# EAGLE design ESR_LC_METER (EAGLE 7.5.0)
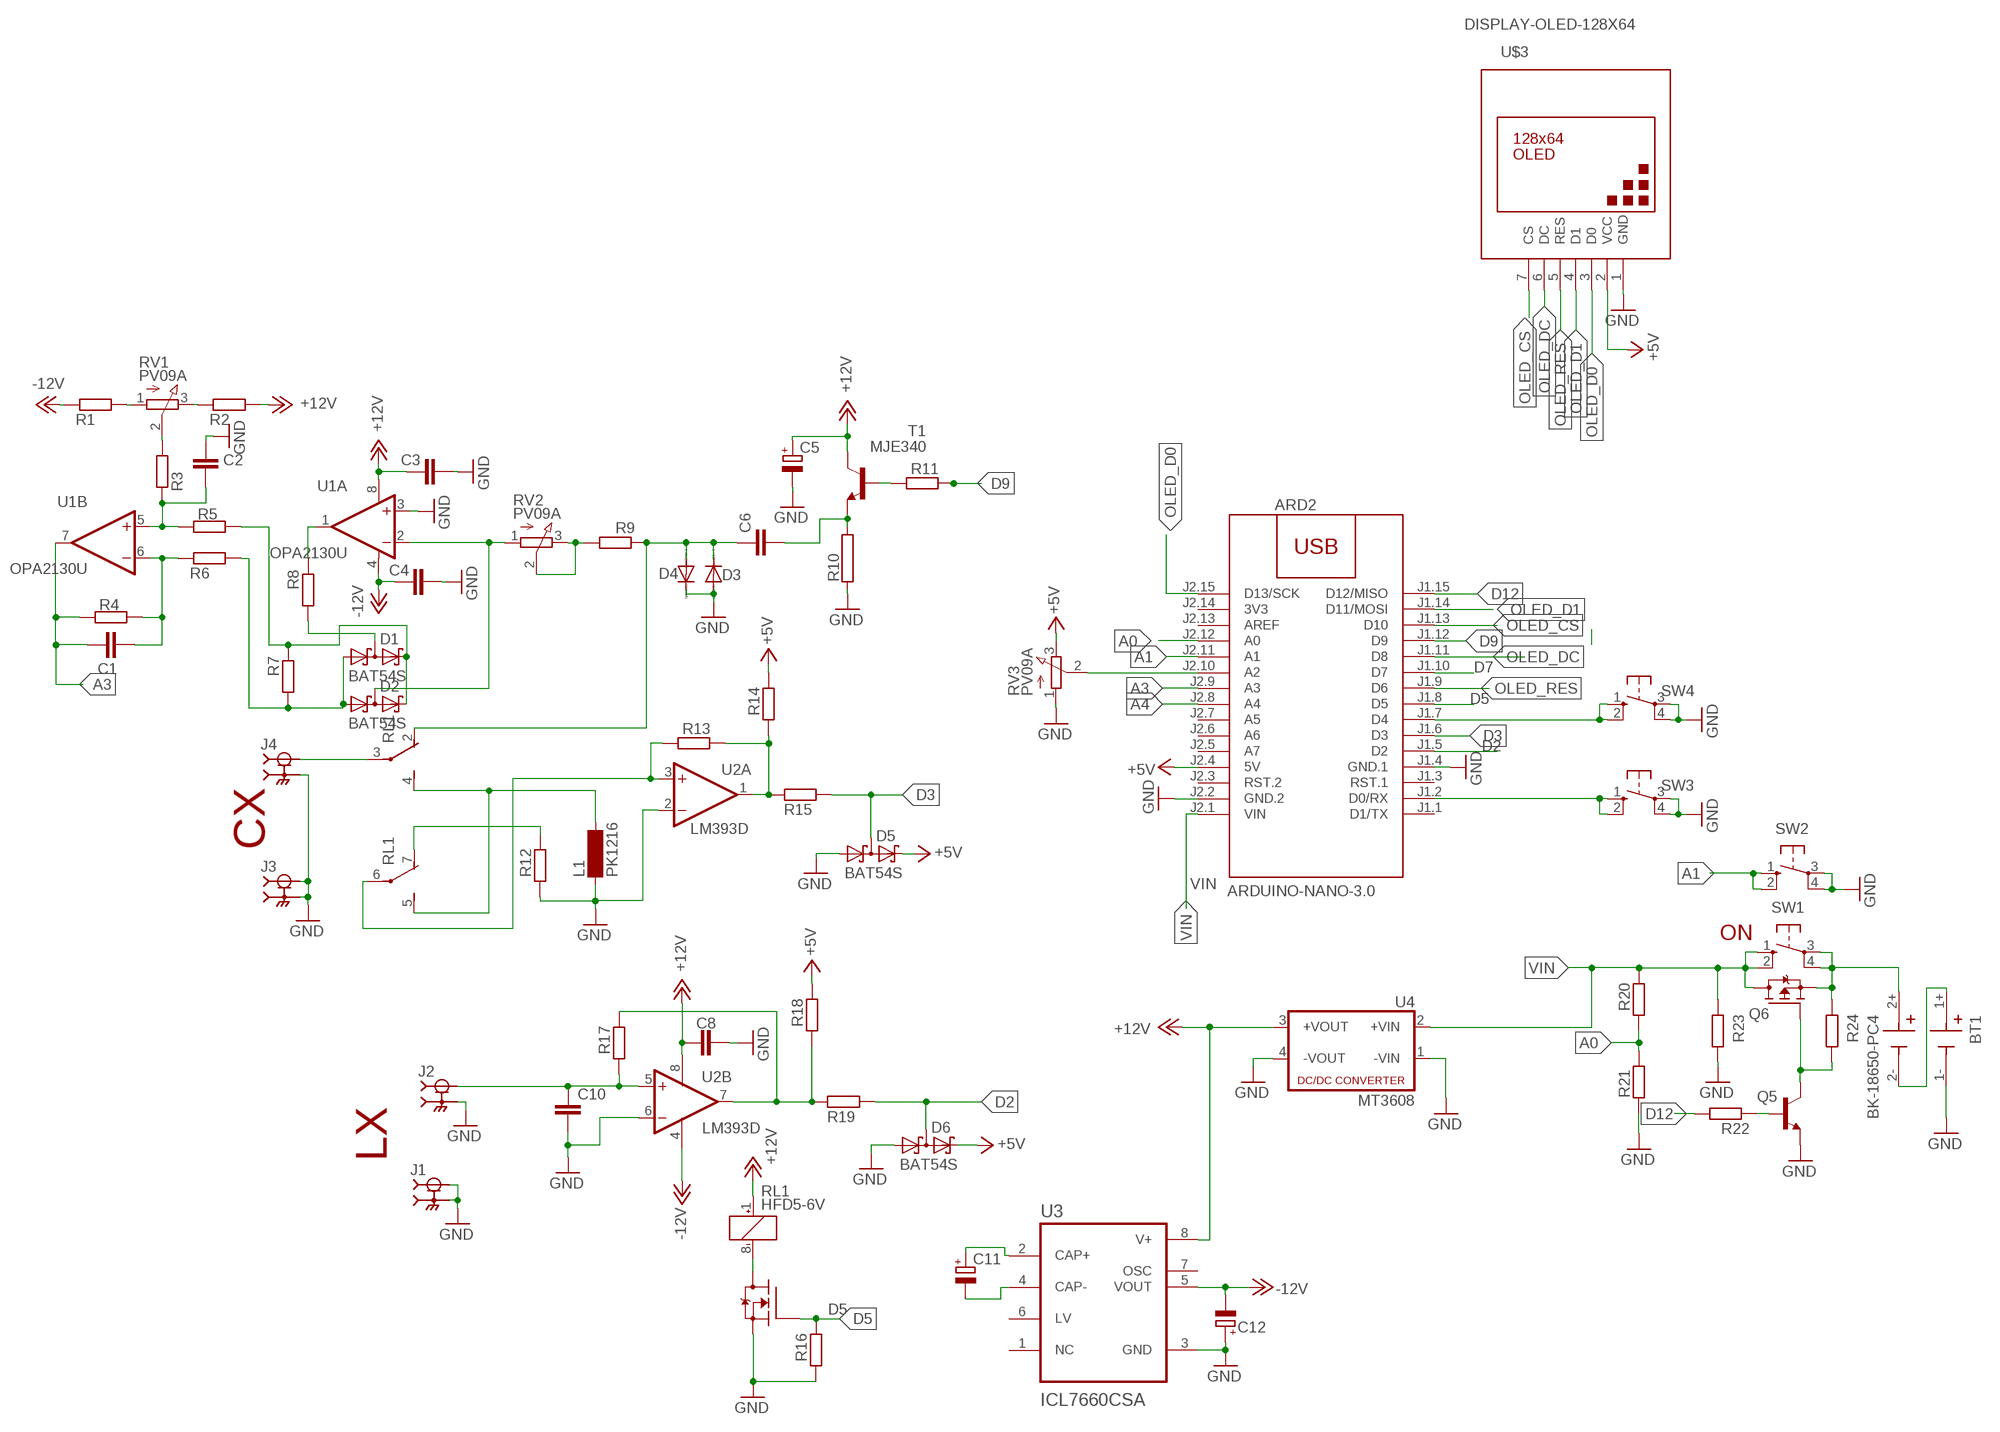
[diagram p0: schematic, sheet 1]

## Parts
ARD2  ARDUINO-NANO-3.0  [ARDUINO-NANO-3.0]
BT1  BK-18650-PC4  [BAT_BK-18650-PC4]
C1  C-EUC0805  [C0805]
C2  C-EUC0805  [C0805]
C3  C-EUC0805  [C0805]
C4  C-EUC0805  [C0805]
C5  CPOL-EUSMCA  [SMC_A]
C6  C-EUC0805  [C0805]
C8  C-EUC0805  [C0805]
C10  C-EUC1206  [C1206]
C11  CPOL-EUSMCA  [SMC_A]
C12  CPOL-EUSMCA  [SMC_A]
D1  BAT54S  [SOT23]
D2  BAT54S  [SOT23]
D3  1N4004  [DO41-10]
D4  1N4004  [DO41-10]
D5  BAT54S  [SOT23]
D6  BAT54S  [SOT23]
J1  BNC7T-J-P-XX-RA-BH1  [SAMTEC_BNC7T-J-P-XX-RA-BH1]
J2  BNC7T-J-P-XX-RA-BH1  [SAMTEC_BNC7T-J-P-XX-RA-BH1]
J3  BNC7T-J-P-XX-RA-BH1  [SAMTEC_BNC7T-J-P-XX-RA-BH1]
J4  BNC7T-J-P-XX-RA-BH1  [SAMTEC_BNC7T-J-P-XX-RA-BH1]
L1  PK1216  BS11  [BS11]
Q3  ZVN3310F  [SOT23]
Q5  BC817-16LT1SMD  [SOT23-BEC]
Q6  STR2P3LLH6  [SOT23]
R1  R-EU_R0805  [R0805]
R2  R-EU_R0805  [R0805]
R3  R-EU_R0805  [R0805]
R4  R-EU_R0805  [R0805]
R5  R-EU_R0805  [R0805]
R6  R-EU_R0805  [R0805]
R7  R-EU_R0805  [R0805]
R8  R-EU_R0805  [R0805]
R9  R-EU_R0805  [R0805]
R10  RAC04  [AC04]
R11  R-EU_R0805  [R0805]
R12  R-EU_R0805  [R0805]
R13  R-EU_R0805  [R0805]
R14  R-EU_R0805  [R0805]
R15  R-EU_R0805  [R0805]
R16  R-EU_R0805  [R0805]
R17  R-EU_R0805  [R0805]
R18  R-EU_R0805  [R0805]
R19  R-EU_R0805  [R0805]
R20  R-EU_R0805  [R0805]
R21  R-EU_R0805  [R0805]
R22  R-EU_R0805  [R0805]
R23  R-EU_R0805  [R0805]
R24  R-EU_R0805  [R0805]
RL1  HFD5-6V  G6J-2P-Y  [G6J-2P-Y]
RV1  PV09A  [PTV09]
RV2  PV09A  [PTV09]
RV3  PV09A  [PTV09]
SW1  10-XX  [B3F-10XX]
SW2  10-XX  [B3F-10XX]
SW3  10-XX  [B3F-10XX]
SW4  10-XX  [B3F-10XX]
T1  MJE340  [TO126]
U1  OPA2130U  [SO08]
U2  LM393D  [SO08]
U3  ICL7660CSA  [SOIC127P600X175-8N]
U4  MT3608  [MT3608]
U$3  DISPLAY-OLED-128X64  [DISPLAY-OLED-128X64]

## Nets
+5V: ARD2.J2.4(5V) D5.2(C2) D6.2(C2) R14.2 R18.2 RV3.3(E) U$3.2(VCC)
+12V: C3.1 C5.+ C8.1 R2.1 RL1.1(1:+) T1.2(C) U1.8(A:V+) U2.8(P:V+) U3.8(V+) U4.3(+VOUT)
-12V: C4.1 C12.- R1.2 U1.4(A:V-) U2.4(P:V-) U3.5(VOUT)
A0: ARD2.J2.12(A0) R20.1 R21.2
A1: ARD2.J2.11(A1) SW2.1(S) SW2.2(S1)
A3: ARD2.J2.9(A3) C1.2 R4.2 U1.7(B:OUT)
A4: ARD2.J2.8(A4)
BAT: BT1.2+ Q6.3(S) R24.2 SW1.3(P) SW1.4(P1)
D2: ARD2.J1.5(D2) D6.3(C1A2) R19.1
D3: ARD2.J1.6(D3) D5.3(C1A2) R15.1
D5: ARD2.J1.8(D5) Q3.2(G) R16.2
D7: ARD2.J1.10(D7)
D9: ARD2.J1.12(D9) R11.2
D12: ARD2.J1.15(D12/MISO) R22.2
GND: ARD2.J1.4(GND.1) ARD2.J2.2(GND.2) BT1.1- C2.2 C3.2 C4.2 C5.- C8.2 C10.2 C12.+ D3.A D4.C D5.1(A1) D6.1(A1) J1.1 J1.S1 J1.S2 J1.S3 J1.S4 J2.S1 J2.S2 J2.S3 J2.S4 J3.1 J3.S1 J3.S2 J3.S3 J3.S4 J4.S1 J4.S2 J4.S3 J4.S4 L1.1 Q3.3(S) Q5.E R10.1 R12.1 R16.1 R21.1 R23.1 RV3.1(A) SW2.3(P) SW2.4(P1) SW3.3(P) SW3.4(P1) SW4.3(P) SW4.4(P1) U1.3(A:+IN) U2.2(A:-IN) U2.6(B:-IN) U3.3(GND) U4.1(-VIN) U4.4(-VOUT) U$3.1(GND)
N$1: ARD2.J1.2(D0/RX) SW3.1(S) SW3.2(S1)
N$2: ARD2.J1.7(D4) SW4.1(S) SW4.2(S1)
N$3: R13.1 RL1.6(3:P) U2.3(A:+IN)
N$4: R13.2 R14.1 R15.2 U2.1(A:OUT)
N$6: C11.+ U3.2(CAP+)
N$7: ARD2.J2.10(A2) RV3.2(S)
N$8: C11.- U3.4(CAP-)
N$9: R17.2 R18.1 R19.2 U2.7(B:OUT)
N$10: Q3.1(D) RL1.8(1:-)
N$11: R11.1 T1.3(B)
N$12: C10.1 J2.1 R17.1 U2.5(B:+IN)
N$13: L1.2 RL1.4(2:S) RL1.5(3:S)
N$14: C6.2 R10.2 T1.1(E)
N$15: R12.2 RL1.7(3:O)
N$16: Q5.C Q6.2(G) R24.1
N$17: J4.1 RL1.3(2:P)
N$18: Q5.B R22.1
N$19: R9.1 RV2.2(S) RV2.3(E)
N$20: C6.1 D3.C D4.A R9.2 RL1.2(2:O)
N$21: D2.3(C1A2) RV2.1(A) U1.2(A:-IN)
N$22: BT1.1+ BT1.2-
N$23: D1.3(C1A2) R8.1
N$24: R8.2 U1.1(A:OUT)
N$25: D1.2(C2) D2.2(C2) R5.1 R7.2
N$26: D1.1(A1) D2.1(A1) R6.1 R7.1
N$27: C2.1 R3.2 R5.2 U1.5(B:+IN)
N$28: C1.1 R4.1 R6.2 U1.6(B:-IN)
N$29: R3.1 RV1.2(S)
N$30: R1.1 RV1.1(A)
N$31: R2.2 RV1.3(E)
OLED_CS: ARD2.J1.13(D10) U$3.7(CS)
OLED_D0: ARD2.J2.15(D13/SCK) U$3.3(D0)
OLED_D1: ARD2.J1.14(D11/MOSI) U$3.4(D1)
OLED_DC: ARD2.J1.11(D8) U$3.6(DC)
OLED_RES: ARD2.J1.9(D6) U$3.5(RES)
VIN: ARD2.J2.1(VIN) Q6.1(D) R20.2 R23.2 SW1.1(S) SW1.2(S1) U4.2(+VIN)
Unconnected: ARD2.J1.1(D1/TX) ARD2.J1.3(RST.1) ARD2.J2.3(RST.2) ARD2.J2.5(A7) ARD2.J2.6(A6) ARD2.J2.7(A5) ARD2.J2.13(AREF) U3.1(NC) U3.6(LV) U3.7(OSC)

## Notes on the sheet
- CX
- ON
- LX

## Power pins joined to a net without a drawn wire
3V3: ARD2.J2.14(3V3)

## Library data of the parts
ARD2 = diy-modules:ARDUINO-NANO-3.0: Arduino Nano 3.0 and compatible devices More details available here: https://www.arduino.cc/en/Main/ArduinoBoardNano Click here to find device on ebay.com
BT1 = BK-18650-PC4:BK-18650-PC4: Battery Holder (Open) 18650 2 Cell PC Pin Check availability; AVAILABILITY: In Stock; CHECK_PRICES: https://www.snapeda.com/parts/BK-18650-PC4/Memory+Protection+Devices/view-part/?ref=eda; DESCRIPTION: Battery Holder (Open) 18650 2 Cell PC Pin; MF: MPD (Memory Protection Devices); MP: BK-18650-PC4; PACKAGE: None; PRICE: None; SNAPEDA_LINK: https://www.snapeda.com/parts/BK-18650-PC4/Memory+Protection+Devices/view-part/?ref=snap
C1-C4 C6 C8 C10 = rcl:C-EU: CAPACITOR, European symbol
C5 C11 C12 = rcl:CPOL-EU: POLARIZED CAPACITOR, European symbol
D1 D2 D5 D6 = diode:BAT54S: Schottky Diodes Pin connection corrected 2011-05-04 Source: Fairchild .. BAT54.pdf
D3 D4 = diode:1N4004: DIODE
J1-J4 = BNC7T-J-P-XX-RA-BH1:BNC7T-J-P-XX-RA-BH1: TRUE 75 OHM RIGHT ANGLE JACK ASSEMBLY Check availability; AVAILABILITY: In Stock; CHECK_PRICES: https://www.snapeda.com/parts/BNC7T-J-P-HN-RA-BH1/Samtec+Inc./view-part/?ref=eda; DESCRIPTION: BNC Connector Jack, Female Socket 75 Ohms Panel Mount, Through Hole, Right Angle Solder; MF: Samtec; MP: BNC7T-J-P-HN-RA-BH1; PACKAGE: None; PRICE: None; PURCHASE-URL: https://www.snapeda.com/api/url_track_click_mouser/?unipart_id=608953&manufacturer=Samtec&part_name=BNC7T-J-P-HN-RA-BH1&search_term=bnc connector; SNAPEDA_LINK: https://www.snapeda.com/parts/BNC7T-J-P-HN-RA-BH1/Samtec+Inc./view-part/?ref=snap
L1 = inductor-neosid:BS: INDUCTOR; OC_FARNELL: unknown; OC_NEWARK: unknown
Q3 = transistor-fet:ZVN3310F
Q5 = transistor-npn:BC817*: NPN Transistor
Q6 = transistor-fet:STR2P3LLH6
R1-R9 R11-R24 = rcl:R-EU_: RESISTOR, European symbol
R10 = resistor-power:R: Power Resitor; OC_FARNELL: unknown; OC_NEWARK: unknown
RL1 = relay:G6J*-2?-Y: Surface-Mounting Signal Relay - G6J-Y 5.7 x 10.6 x 9 mm Source: http://www.omroncomponents.eu/ .. K125-E2-02-X.pdf; MF: OMRON COMPONENTS USA; MPN: G6J-2P-Y-DC12; OC_FARNELL: unknown; OC_NEWARK: 70J9830
RV1-RV3 = pot:PV09A
SW1-SW4 = switch-omron:10-XX: OMRON SWITCH; MPN: B3F-1000; OC_FARNELL: 176432; OC_NEWARK: 36M3542
T1 = transistor:MJE340: NPN TRANSISTOR
U1 = burr-brown:OPA2130: Operational Amplifier; MF: TEXAS INSTRUMENTS; MPN: OPA2130UA; OC_FARNELL: 1459554; OC_NEWARK: 35C1841
U2 = linear:LM393: COMPARATOR
U3 = ICL7660CSA:ICL7660CSA: Check availability; AVAILABILITY: In Stock; CHECK_PRICES: https://www.snapeda.com/parts/ICL7660CSA/Analog+Devices/view-part/?ref=eda; DESCRIPTION: Charge Pump Switching Regulator IC Positive or Negative Fixed -Vin, nVin, Vin/2 1 Output 20mA 8-SOIC (0.154, 3.90mm Width); MF: Analog Devices; MP: ICL7660CSA; PACKAGE: SOIC-8 Maxim; PRICE: None; SNAPEDA_LINK: https://www.snapeda.com/parts/ICL7660CSA/Analog+Devices/view-part/?ref=snap
U4 = dc-dc-converter:MT3608: DC DC Up Converter
U$3 = diy-modules:DISPLAY-OLED-128X64: 128x64 Dot Matrix OLED Module based on SSD1306 chip Variant with SPI interface More details available here: http://www.instructables.com/id/How-to-use-OLED-display-arduino-module/ SSD1306 datasheet: https://cdn-shop.adafruit.com/datasheets/SSD1306.pdf Click here to find device on ebay.com Note: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

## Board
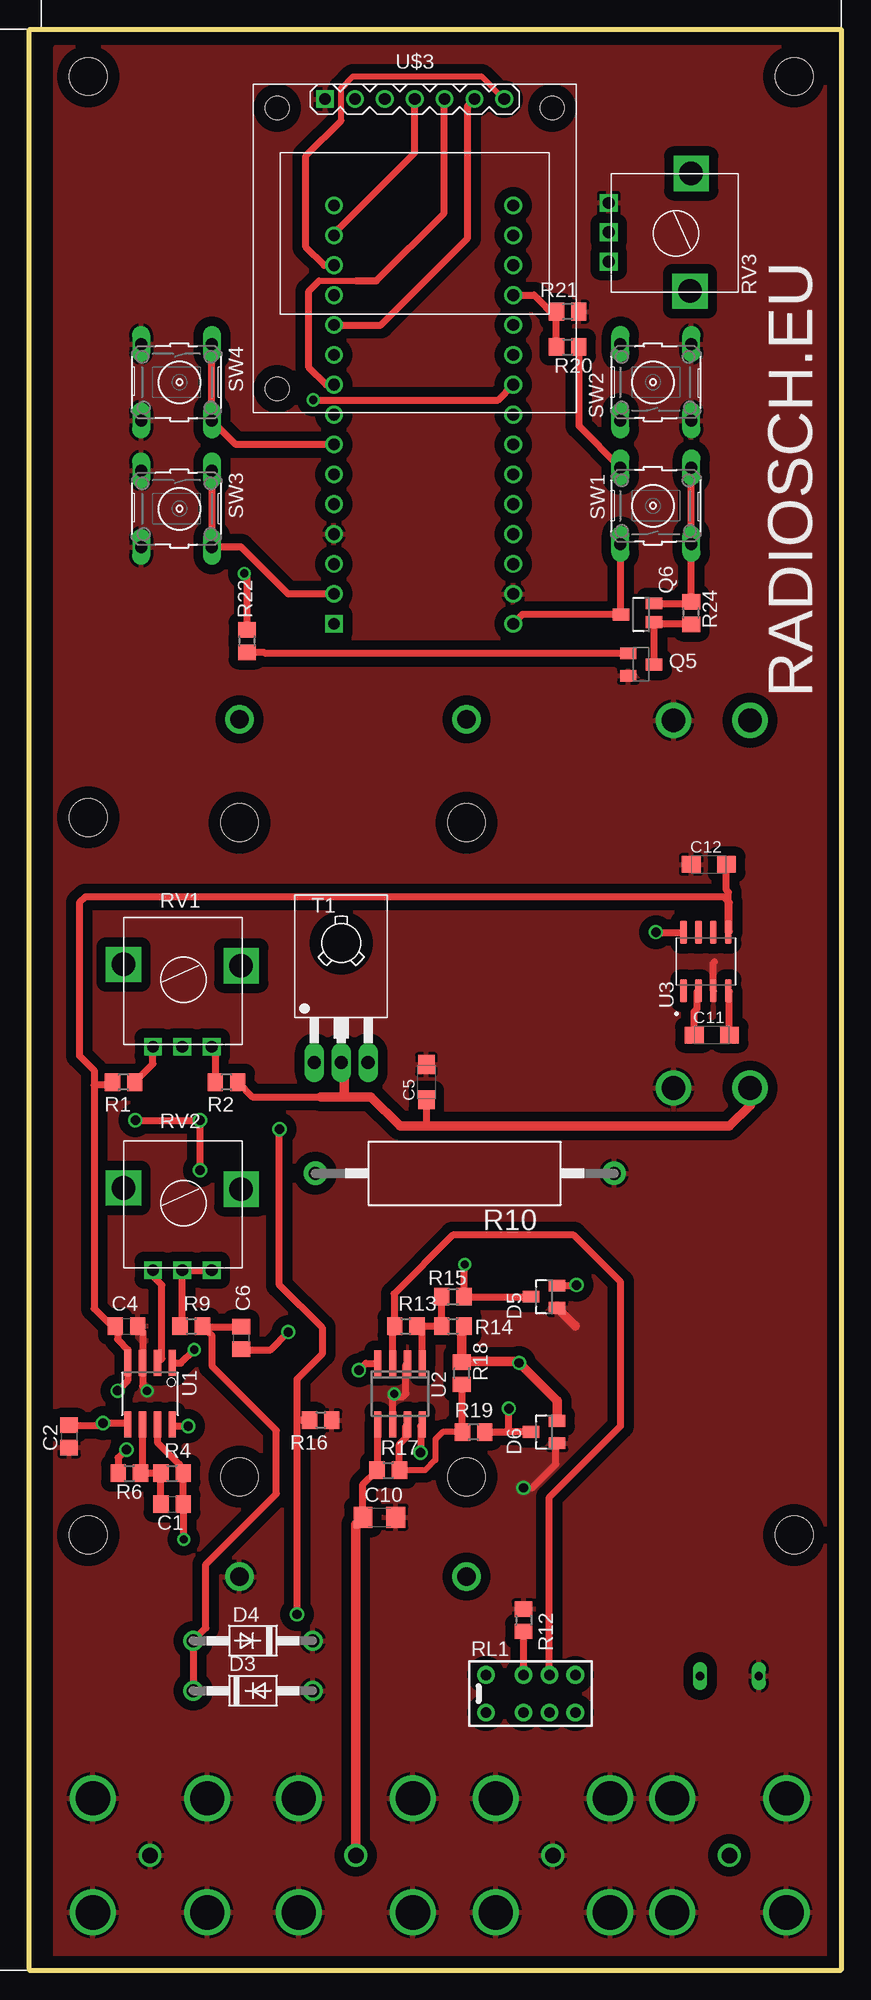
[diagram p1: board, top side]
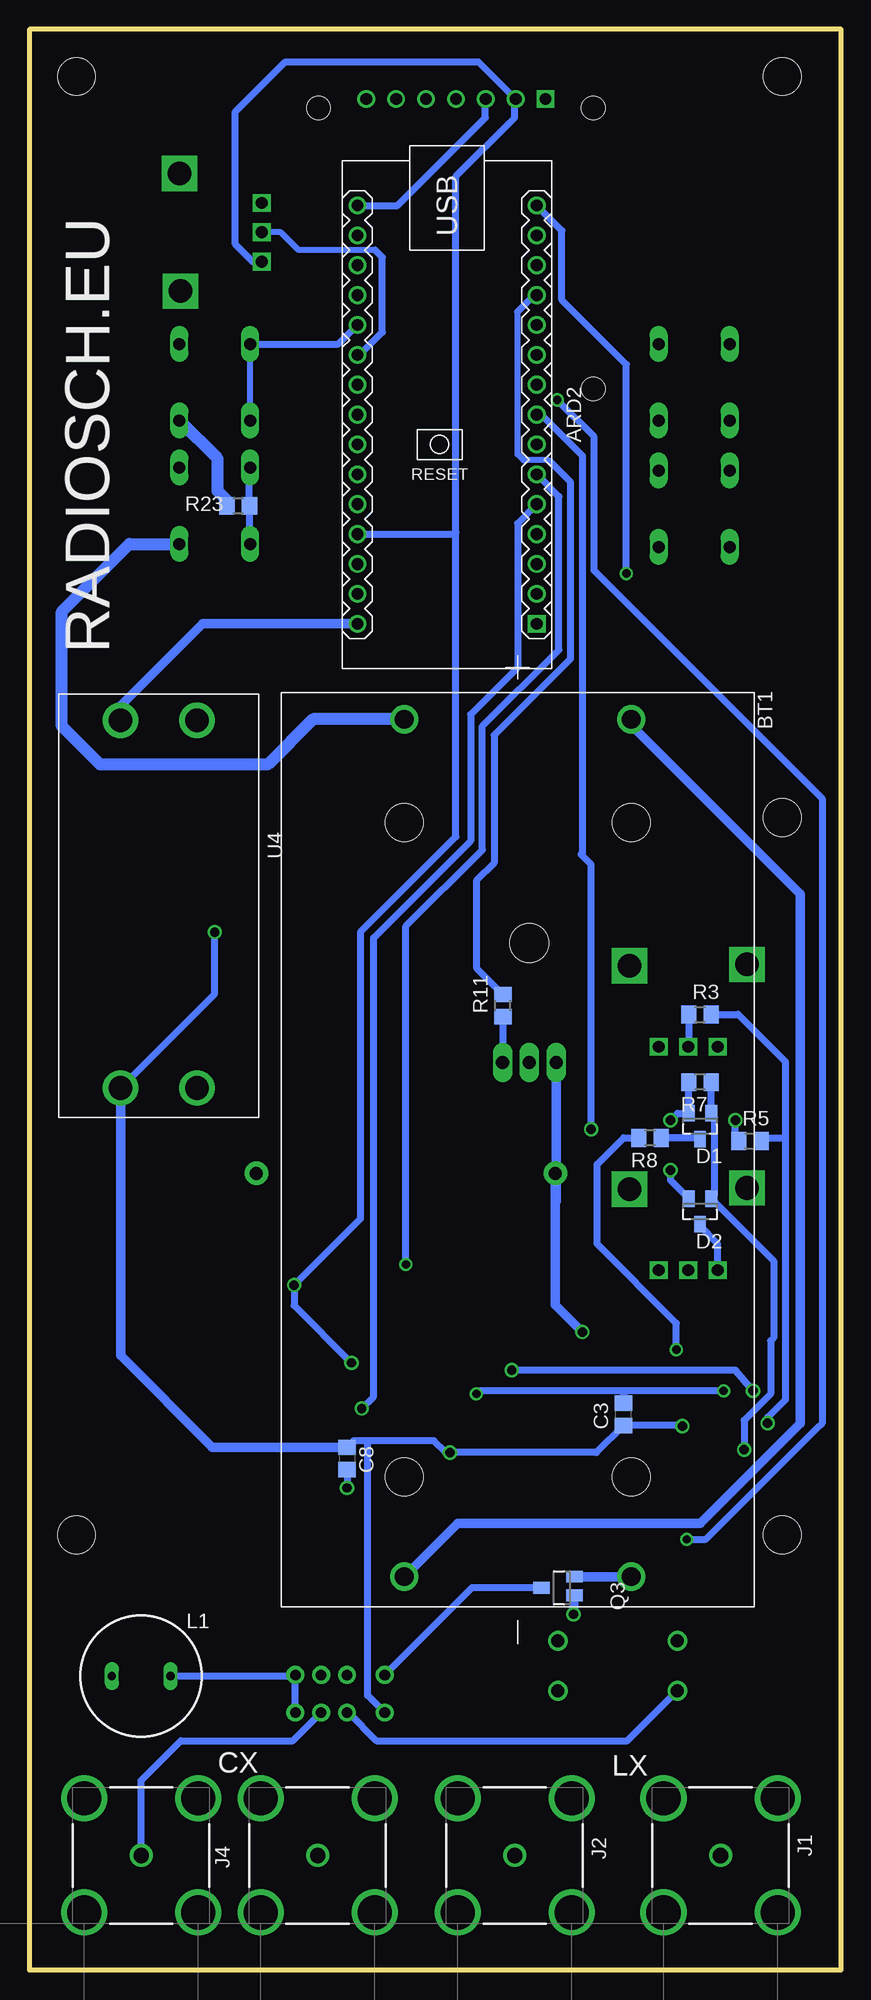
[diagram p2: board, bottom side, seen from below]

Size 69 x 165 mm. Coordinates in mm from the lower left corner, seen from the top.
Outline: 0,0 0,165 69,165 69,0 0,0
Copper layers (1*16): Top 0.035mm / dielectric 1.5mm / Bottom 0.035mm
Design rules "default *": minimum track width 10mil, minimum drill 15mil, track to track 6mil, track to pad 6mil, pad to pad 6mil, via to via 6mil, smd to smd 4mil, copper to edge 40mil, drill to drill 8mil, minimum pad ring 10mil, minimum via ring 8mil, stop-mask expansion 4mil, vias tented up to drill 0mil, thermal gap 10mil
Holes 3.2 mm at 5,161 65,161 5,98 5,37 65,37

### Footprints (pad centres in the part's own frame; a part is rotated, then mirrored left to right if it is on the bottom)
ARDUINO-NANO-3.0 = drill 1 square: J1.1 17.78,7.62 | drill 1: J1.2 15.24,7.62; J1.3 12.7,7.62; J1.4 10.16,7.62; J1.5 7.62,7.62; J1.6 5.08,7.62; J1.7 2.54,7.62; J1.8 0,7.62; J1.9 -2.54,7.62; J1.10 -5.08,7.62; J1.11 -7.62,7.62; J1.12 -10.16,7.62; J1.13 -12.7,7.62; J1.14 -15.24,7.62; J1.15 -17.78,7.62; J2.1 17.78,-7.62; J2.2 15.24,-7.62; J2.3 12.7,-7.62; J2.4 10.16,-7.62; J2.5 7.62,-7.62; J2.6 5.08,-7.62; J2.7 2.54,-7.62; J2.8 0,-7.62; J2.9 -2.54,-7.62; J2.10 -5.08,-7.62; J2.11 -7.62,-7.62; J2.12 -10.16,-7.62; J2.13 -12.7,-7.62; J2.14 -15.24,-7.62; J2.15 -17.78,-7.62
BAT_BK-18650-PC4 = drill 1.6: 1+ -36.6,9.65; 1- 36.3,9.65; 2+ -36.6,-9.65; 2- 36.3,-9.65 | hole 3.2: -27.81,-9.65; -27.81,9.65; 27.81,-9.65; 27.81,9.65
C0805 = smd 1.3 x 1.5: 1 -0.95,0; 2 0.95,0
SMC_A = smd 1.6 x 1.4: + -1.5,0; - 1.5,0
C1206 = smd 1.6 x 1.8: 1 -1.4,0; 2 1.4,0
SOT23 = smd 1 x 1.4: 1 -0.95,-1.1; 2 0.95,-1.1; 3 0,1.1
DO41-10 = drill 1.118: A 5.08,0; C -5.08,0
SAMTEC_BNC7T-J-P-XX-RA-BH1 = drill 1.3: 1 0,0 | drill 2.9: S1 -4.85,4.85; S2 4.85,4.85; S3 4.85,-4.85; S4 -4.85,-4.85
BS11 = drill 0.7 long: 1 -2.5,0; 2 2.5,0
SOT23' = smd 1 x 1.4: 1 0,1.735; 2 -0.632,-1.1; 3 0.95,-1.1
SOT23-BEC = smd 1 x 1.4: B -0.95,-1.1; C 0,1.1; E 0.95,-1.1
R0805 = smd 1.3 x 1.5: 1 -0.95,0; 2 0.95,0
AC04 = drill 1.1 pad 2: 1 -12.7,0; 2 12.7,0
G6J-2P-Y = drill 0.9 pad 1.5: 1 -3.2,-1.6; 2 0,-1.6; 3 2.2,-1.6; 4 4.4,-1.6; 5 4.4,1.6; 6 2.2,1.6; 7 0,1.6; 8 -3.2,1.6
PTV09 = drill 1 square: 1 -2.5,0; 2 0,0; 3 2.5,0 | drill 2 square: P$4 -5,7; P$5 5,6.9
B3F-10XX = drill 1.016 long: 1 -3.251,2.761; 2 3.251,2.761; 3 -3.251,-3.261; 4 3.251,-3.261
TO126 = drill 1.118 long: 1 -2.286,-5.08; 2 0,-5.08; 3 2.286,-5.08 | hole 3.302: 0,5.08
SO08 = smd 0.61 x 2.21: 1 -1.905,-2.616; 2 -0.635,-2.616; 3 0.635,-2.616; 4 1.905,-2.616; 5 1.905,2.616; 6 0.635,2.616; 7 -0.635,2.616; 8 -1.905,2.616
SO08' = smd 0.6 x 2.2: 1 -1.905,-2.6; 2 -0.635,-2.6; 3 0.635,-2.6; 4 1.905,-2.6; 5 1.905,2.6; 6 0.635,2.6; 7 -0.635,2.6; 8 -1.905,2.6
SOIC127P600X175-8N = smd 1.97 x 0.59: 1 -2.475,1.905; 2 -2.475,0.635; 3 -2.475,-0.635; 4 -2.475,-1.905; 5 2.475,-1.905; 6 2.475,-0.635; 7 2.475,0.635; 8 2.475,1.905
MT3608 = drill 2: 1 2.25,11.75; 2 2.25,5.25; 3 33.5,5.25; 4 33.5,11.75
DISPLAY-OLED-128X64 = drill 1 square: 1 -7.62,12.7 | drill 1: 2 -5.08,12.7; 3 -2.54,12.7; 4 0,12.7; 5 2.54,12.7; 6 5.08,12.7; 7 7.62,12.7 | hole 2: -11.684,11.938; 11.684,11.938; -11.684,-11.938

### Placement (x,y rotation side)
ARD2  33.5,132.25 270 bottom
BT1  27.5,69.75 270 bottom
C1  12.12,39.62 0 top
C2  3.38,45.38 270 top
C3  18.5,47.25 90 bottom
C4  8.25,54.75 0 top
C5  33.75,75.5 90 top
C6  18,53.75 270 top
C8  42,43.5 270 bottom
C10  29.75,38.5 0 top
C11  58,79.5 0 top
C12  57.75,94 0 top
D1  12,71.75 180 bottom
D2  12,64.5 180 bottom
D3  19,23.75 0 top
D4  19,28 180 top
D5  43.75,57.25 90 top
D6  43.75,45.75 90 top
J1  10.25,9.75 180 bottom
J2  27.75,9.75 180 bottom
J3  44.5,9.75 180 bottom
J4  59.5,9.75 180 bottom
L1  59.5,25 0 bottom
Q3  ZVN3310F  [SOT23']  23.75,32.5 90 bottom
Q5  52,111 270 top
Q6  STR2P3LLH6  [SOT23']  52,115.25 90 top
R1  8,75.5 180 top
R2  16.75,75.5 180 top
R3  12,81.25 0 bottom
R4  12.12,42.25 0 top
R5  7.75,70.5 0 bottom
R6  8.5,42.25 0 top
R7  12,75.5 180 bottom
R8  16.25,70.75 180 bottom
R9  13.75,54.75 0 top
R10  37,67.75 180 top
R11  28.75,82 90 bottom
R12  42,29.75 270 top
R13  32,54.75 0 top
R14  36,54.75 0 top
R15  36,57.25 180 top
R16  24.75,46.75 180 top
R17  30.5,42.5 0 top
R18  36.75,50.75 90 top
R19  37.75,45.75 180 top
R20  45.75,138 0 top
R21  45.75,141 180 top
R22  18.5,113 90 top
R23  51.25,124.5 0 bottom
R24  56.25,115.38 90 top
RL1  42,23.5 0 top
RV1  13,78.5 0 top
RV2  13,59.5 0 top
RV3  49.25,147.75 270 top
SW1  53,124.5 90 top
SW2  53,135 90 top
SW3  12.75,124.25 270 top
SW4  12.75,135 270 top
T1  26.5,82.25 0 top
U1  10.25,49 180 top
U2  LM393D  [SO08']  31.5,49 180 top
U3  57.5,85.75 90 top
U4  66.5,108.5 270 bottom
U$3  32.75,146.38 0 top

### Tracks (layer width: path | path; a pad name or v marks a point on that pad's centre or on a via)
+5V  (via drill 0.8)
  Top 0.61: D5.2 46.45,58.2 v46.5,58.25 | v41.62,51.62 40.62,51.62 40.5,51.75
  Top 0.813: D6.2 44.85,48.4 v41.62,51.62 41.5,51.75 40.5,51.75 36.8,51.75 R18.2 36.75,54.55 R14.2
  Bottom 0.61: v41.62,51.62 46.5,56.5 v46.5,58.25 40.88,63.88 40.88,88.25 32.75,96.38 32.75,122.25 | 32.75,122.25 32.75,152.5 27.75,157.5 27.75,159 U$3.2 30.84,162.25 47.25,162.25 51.5,158 51.5,146.75 50,145.25 RV3.3 | ARD2.J2.4 32.91,122.09 32.75,122.25
+12V  (via drill 0.8)
  Top 0.61: R2.1 18.95,74.25 24.75,74.25 | 26.5,76 T1.2 | v53.25,88.25 53.27,88.22 U3.8 | U1.8 12.29,46.25 v13.5,46.25 | U2.8 33.25,46.24 v33.25,44 | C5.+ 33.75,72 34,71.75
  Top 0.813: 24.75,74.25 26.75,74.25 | 26.75,74.25 29,74.25 31.5,71.75 34,71.75 59.5,71.75 61.25,73.5 U4.3 | 26.5,76 26.75,75.75 26.75,74.25
  Bottom 0.61: U4.3 53.25,83 v53.25,88.25 | v13.5,46.25 13.55,46.3 C3.1 20.8,44 v33.25,44 33.62,44 34.62,45 40.5,45 | 41.95,44.45 C8.1 | RL1.1 40.25,23.35 40.25,44.75 40.5,45 | 41.95,44.5 C8.1 | 40.5,45 41.45,45 C8.1
  Bottom 0.813: U4.3 61.25,52.25 53.45,44.45 C8.1
-12V  (via drill 0.8)
  Top 0.61: 5.5,75.25 5.5,76.5 4.25,77.75 4.25,90.75 4.75,91.25 59,91.25 59.5,90.75 59.5,88.32 U3.5 59.41,91.66 59.25,91.81 C12.- | 5.5,75.25 5.5,56.25 7,54.75 C4.1 7.25,54.7 7.5,54.45 7.5,53.62 8.38,52.75 8.38,51.65 U1.4 8.35,50.09 v7.5,49.25 | R1.2 6.8,75.25 5.5,75.25 | v28,51 28.6,51.6 U2.4
  Bottom 0.61: v7.5,49.25 9,51 v28,51
A0
  Top 0.61: R20.1 44.8,140.5 | 44.8,140.5 R21.2 | ARD2.J2.12 42.89,142.41 44.8,140.5
A1
  Bottom 0.5: SW2.1 SW2.2
  Bottom 0.61: SW2.2 42.74,138.25 ARD2.J2.11
A3  (via drill 0.7)
  Top 0.61: U1.7 10.88,44.87 12.75,43 12.75,42.58 R4.2 C1.2 13.07,36.67 v13.12,36.62 | v24.12,133.5 39.83,133.5 ARD2.J2.9
  Bottom 0.61: v13.12,36.62 11.5,36.62 2.31,45.81 2.12,46 1.62,46.5 1.62,99.62 21,119 21,130.38 v24.12,133.5
BAT
  Top 0.61: Q6.3 56.12,116.2 R24.2 56.25,121.24 SW1.3 SW1.4
  Bottom 1.016: BT1.2+ 44.9,106.35 48.75,102.5 63,102.5 66.25,105.75 66.25,115.5 60.5,121.25 SW1.3
D2  (via drill 0.8)
  Top 0.61: D6.3 40.5,45.75 | R19.1 40.5,45.75 | 40.5,45.75 40.75,46 v40.75,47.75
  Bottom 0.61: v40.75,47.75 39.75,48.75 39.75,87.75 31.5,96 31.5,106.75 27.5,110.75 27.5,123 ARD2.J1.5
D3  (via drill 0.7)
  Top 0.61: D5.3 R15.1 36.95,59.95 v37,60
  Bottom 0.61: v37,60 37,88.75 30.5,95.25 30.5,105.75 24,112.25 24,125.29 ARD2.J1.6
D5  (via drill 0.8)
  Top 0.61: v21.25,71.5 21.25,58.25 24.88,54.62 24.88,52.38 22.75,50.25 22.75,47 | v22.75,30.25 22.75,47 | R16.2 23,46.75 22.75,47
  Bottom 0.61: v21.25,71.5 21.25,94 22.12,94.88 22,95 22,128.75 25.5,132.25 ARD2.J1.8
  Bottom 0.813: Q3.2 22.75,31.77 v22.75,30.25
D9
  Bottom 0.5: 24.75,128.25 24.88,128.38 27,128.38 27.5,128.88 27.5,141
  Bottom 0.61: ARD2.J1.12 26.09,142.41 27.5,141 | 24.75,128.25 23,126.5 23,111.5 29.5,105 29.5,94.12 31,92.62 31,85.2 R11.2
D12  (via drill 0.7)
  Top 0.61: R22.2 18.5,118.5 v18.25,118.75
  Bottom 0.61: ARD2.J1.15 23.75,147.9 23.75,142 18.25,136.5 v18.25,118.75
GND  (via drill 0.7, 0.8)
  Top 0.61: U2.2 32,51.47 32,49 31.75,48.75 30.75,48.75 30.86,48.63 U2.6 30.86,48.87 v31,49 | v42,41 42.75,41 44.75,43 44.75,44.7 D6.1 | U3.3 58.13,85.64 58.25,85.75 | C4.2 9.62,54.34 U1.3 9.62,49.63 v10,49.25
  Top 0.813: 46.4,54.75 D5.1
  Bottom 0.61: C8.2 v42,41 | v10,49.25 18.25,49.25 | 18.25,49.25 30.75,49.25 v31,49 | C3.2 18.5,49 18.25,49.25
  Bottom 0.813: Q3.3 BT1.1-
  Bottom 1.016: R23.1 52.2,124.95 53,125.75 53,128.49 SW2.3
  pour Top (isolate 0.813): 2.25,163.5 68,163.5 68,1 2.25,1
N$1
  Top 0.61: ARD2.J1.2 22,117 18,121 SW3.2 SW3.1
N$2
  Top 0.61: ARD2.J1.7 17.55,129.71 SW4.2 SW4.1
N$3
  Top 0.61: U2.3 30.86,54.25 | 30.86,54.25 30.86,54.56 R13.1 | RL1.6 44.2,40.2 50.25,46.25 50.25,58.5 46.25,62.5 36,62.5 31,57.5 31,54.38 30.86,54.25
N$4
  Top 0.61: R13.2 33.5,54.75 | 33.5,54.75 R14.1 R15.2 | U2.1 33.41,54.66 33.5,54.75
N$6
  Top 0.61: C11.+ 56.5,81.5 56.75,81.75 56.75,83.16 U3.2
N$7
  Bottom 0.5: 39.62,146.25 46.12,146.25 47.62,147.75 RV3.2
  Bottom 0.61: ARD2.J2.10 40.92,137.33 39,139.25 39,145.62 39.62,146.25
N$8
  Top 0.61: C11.- 59.5,83.18 U3.4
N$9
  Top 0.5: R19.2 35.12,45.75 34.5,45.12 34.5,43.38 33.62,42.5 R17.2
  Top 0.61: R17.2 31.45,44.7 32,45.25 32,46.27 U2.7 | R19.2 36.8,49.75 R18.1
N$10
  Bottom 0.61: Q3.1 31.4,32.5 RL1.8
N$11
  Bottom 0.61: R11.1 28.75,77.21 T1.3
N$12
  Top 0.61: U2.5 29.59,42.5 R17.1 28.35,41.3 C10.1
  Top 0.813: J2.1 27.75,37.9 C10.1
N$13
  Bottom 0.61: L1.2 46.5,25 RL1.5 RL1.4
N$14  (via drill 0.8)
  Top 0.61: C6.2 18.05,52.75 20.5,52.75 v22,54.25
  Bottom 0.813: v22,54.25 24.3,56.55 R10.2 24.21,65.34 T1.1
N$15
  Top 0.61: RL1.7 R12.2
N$16
  Top 0.61: Q5.C Q6.2 53.29,114.42 R24.1
N$17
  Bottom 0.61: J4.1 59.5,16.12 56.12,19.5 46.6,19.5 RL1.3
N$18
  Top 0.61: Q5.B 20.05,111.95 20,112 18.55,112 R22.1
N$19
  Top 0.61: R9.1 13,54.95 RV2.2 RV2.3
N$20
  Top 0.61: R9.2 14.75,54.7 | 14.75,54.7 C6.1 | 14.75,54.7 15.5,53.95 15.5,51.38 21,45.88 21,40.5 15,34.5 15,29.08 D4.A D3.C
  Bottom 0.61: RL1.2 41.9,21.9 39.5,19.5 18.17,19.5 D3.C
N$21
  Top 0.61: U1.2 11.25,51.98 11.25,58.25 10.5,59 RV2.1
  Bottom 0.61: RV2.1 10.5,61.75 12,63.25 D2.3
N$22
  Bottom 0.813: BT1.2- 32.6,38 12,38 3.5,46.5 3.5,91.5 17.85,105.85 BT1.1+
N$23
  Bottom 0.61: D1.3 12.1,70.75 R8.1
N$24  (via drill 0.7)
  Top 0.61: U1.1 12.87,51.62 v14,52.75
  Bottom 0.61: v14,52.75 14,55 20.75,61.75 20.75,68.5 18.5,70.75 R8.2
N$25  (via drill 0.8)
  Top 0.61: v14.5,68 v14.5,72.25 v9,72.25
  Bottom 0.61: D2.2 14.5,67.15 v14.5,68 | v14.5,72.25 13.9,72.85 D1.2 R7.2 | R5.1 9,70.8 v9,72.25
N$26  (via drill 0.8)
  Top 0.61: v8.25,44.25 7.55,43.55 R6.1
  Bottom 0.61: R7.1 D1.1 11.05,72.8 10.75,72.5 10.75,65.9 D2.1 5.75,60.3 5.75,53.75 6,53.5 6,49 8.25,46.75 v8.25,44.25
N$27  (via drill 0.8)
  Top 0.61: U1.5 8.23,46.5 v6.25,46.5 6.08,46.33 C2.1
  Bottom 0.61: R3.2 8.75,81.25 4.75,77.25 4.75,70.75 | 4.75,70.75 4.75,48.5 6.25,47 v6.25,46.5 | R5.2 6.55,70.75 4.75,70.75
N$28
  Top 0.61: U1.6 9.62,42.41 R6.2 R4.1 C1.1
N$29
  Bottom 0.61: R3.1 12.95,78.55 RV1.2
N$30
  Top 0.61: R1.1 10.5,77.05 RV1.1
N$31
  Top 0.61: RV1.3 15.8,78.2 R2.2
OLED_CS
  Top 0.5: 26.5,157.25 26.5,160 27.5,161 38.45,161 U$3.7
  Top 0.61: ARD2.J1.13 25.05,144.95 23.5,146.5 23.5,154.25 26.5,157.25
OLED_D0
  Bottom 0.61: ARD2.J2.15 37.72,150.03 30.25,157.5 30.25,159.03 U$3.3
OLED_D1
  Top 0.61: ARD2.J1.14 25.88,147.63 32.75,154.5 U$3.4
OLED_DC
  Top 0.61: ARD2.J1.11 29.87,139.87 37.25,147.25 37.25,158.5 U$3.6
OLED_RES
  Top 0.5: 24.62,143.62 27.75,143.62
  Top 0.61: ARD2.J1.9 25.21,134.79 23.75,136.25 23.75,142.75 24.62,143.62 | 27.75,143.62 29.5,143.62 35.25,149.38 35.25,159.03 U$3.5
VIN
  Top 0.61: SW1.1 50.27,121.22 Q6.1 41.9,115.25 ARD2.J2.1 | R20.2 46.7,131.29 SW1.2
  Bottom 0.61: SW1.1 50.3,121.31 R23.2 50.3,127.69 SW1.2
  Bottom 0.813: U4.2 61.25,107.5 54.25,114.5 41.15,114.5 ARD2.J2.1

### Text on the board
tPlace: RADIOSCH.EU
bPlace: RADIOSCH.EU | CX | LX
